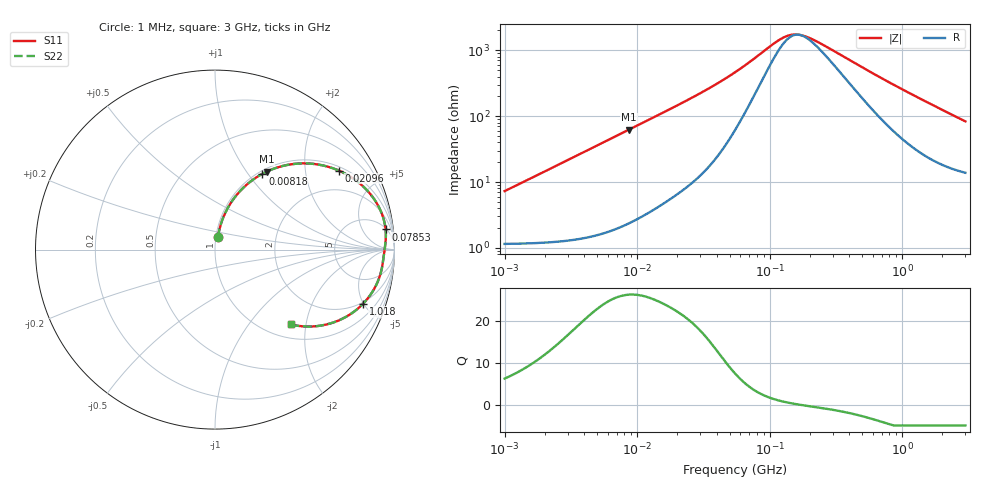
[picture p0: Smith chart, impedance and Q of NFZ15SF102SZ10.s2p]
! NFZ15SF102SZ10
# Hz S RI R 50
!Freq.(Hz) S11(Real) S11(Imag) S21(Real) S21(Imag) S12(Real) S12(Imag) S22(Real) S22(Imag)
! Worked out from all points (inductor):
!   401 points, 1 MHz to 3 GHz, reference 50 ohm
!   read as one part in series: L = 1.14 uH near 1.041 MHz
!   highest Q = 26.4 at 8.686 MHz (marker M1), where L = 1.14 uH
!   self-resonance near 166.9 MHz
!   S11 on the Smith chart (normalised r, x): 1 MHz: 1.02, +0.14; 8.18 MHz: 1.04, +1.17; 20.96 MHz: 1.14, +3.04; 78.53 MHz: 6, +15; 1.018 GHz: 1.87, -4.95; 3 GHz: 1.28, -1.64
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1000000  0.0163 0.0698  0.9837 -0.0698  0.9837 -0.0698  0.0163 0.0698
2014875  0.0316 0.1384  0.9684 -0.1384  0.9684 -0.1384  0.0316 0.1384
3823119  0.081 0.2487  0.919 -0.2487  0.919 -0.2487  0.081 0.2487
5705239  0.1538 0.3407  0.8462 -0.3407  0.8462 -0.3407  0.1538 0.3407
8179831  0.2644 0.4224  0.7356 -0.4224  0.7356 -0.4224  0.2644 0.4224
8686058  0.2874 0.434  0.7126 -0.434  0.7126 -0.434  0.2874 0.434
1.149534e7  0.4091 0.4728  0.5909 -0.4728  0.5909 -0.4728  0.4091 0.4728
1.461624e7  0.5245 0.4796  0.4755 -0.4796  0.4755 -0.4796  0.5245 0.4796
2.095589e7  0.6905 0.4401  0.3095 -0.4401  0.3095 -0.4401  0.6905 0.4401
3.387922e7  0.8525 0.3244  0.1475 -0.3244  0.1475 -0.3244  0.8525 0.3244
5.477226e7  0.9318 0.194  0.0682 -0.194  0.0682 -0.194  0.9318 0.194
7.852918e7  0.9504 0.1124  0.0496 -0.1124  0.0496 -0.1124  0.9504 0.1124
1.125904e8  0.9509 0.0506  0.0491 -0.0506  0.0491 -0.0506  0.9509 0.0506
1.375402e8  0.9482 0.0234  0.0518 -0.0234  0.0518 -0.0234  0.9482 0.0234
1.680187e8  0.945 -0.000807  0.055 0.000807  0.055 0.000807  0.945 -0.000807
2.094008e8  0.9416 -0.0259  0.0584 0.0259  0.0584 0.0259  0.9416 -0.0259
4.75755e8  0.9209 -0.1389  0.0791 0.1389  0.0791 0.1389  0.9209 -0.1389
8.005644e8  0.8701 -0.246  0.1299 0.246  0.1299 0.246  0.8701 -0.246
1.017911e9  0.8243 -0.3023  0.1757 0.3023  0.1757 0.3023  0.8243 -0.3023
1.347129e9  0.7469 -0.3646  0.2531 0.3646  0.2531 0.3646  0.7469 -0.3646
1.855641e9  0.6274 -0.4156  0.3726 0.4156  0.3726 0.4156  0.6274 -0.4156
3e9  0.422 -0.4168  0.578 0.4168  0.578 0.4168  0.422 -0.4168
